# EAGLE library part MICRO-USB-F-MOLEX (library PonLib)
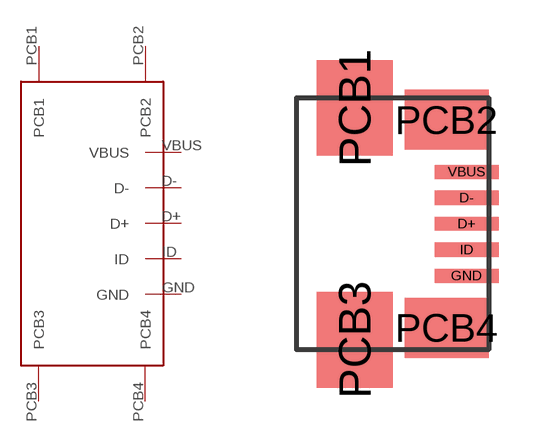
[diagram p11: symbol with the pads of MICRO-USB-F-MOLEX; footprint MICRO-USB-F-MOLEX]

Designator prefix -

## MICRO-USB-F-MOLEX  [MICRO-USB-F-MOLEX]
D+  D+
D-  D-
GND  GND
ID  ID
PCB1  PCB1
PCB2  PCB2
PCB3  PCB3
PCB4  PCB4
VBUS  VBUS

## Footprint MICRO-USB-F-MOLEX (pad centres in mm)
smd 1.6 x 0.35: D+ 2.8,0; D- 2.8,0.65; GND 2.8,-1.3; ID 2.8,-0.65; VBUS 2.8,1.3
smd 1.9 x 2.4: PCB1 0,2.9; PCB3 0,-2.9
smd 2.1 x 1.5: PCB2 2.3,2.6; PCB4 2.3,-2.6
